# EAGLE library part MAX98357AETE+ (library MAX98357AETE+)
MAXIM INTEGRATED PRODUCTS - MAX98357AETE+ - AMPLIFIER, CLASS-D, 1-CH, 3.2W, TQFN-16 Source: Datasheet
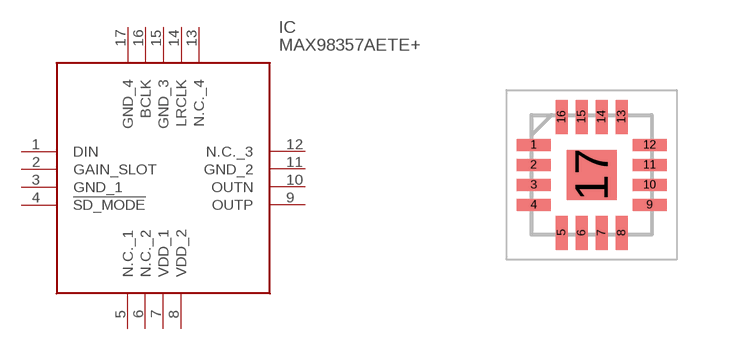
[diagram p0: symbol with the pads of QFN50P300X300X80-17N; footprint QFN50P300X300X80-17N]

Designator prefix IC

## MAX98357AETE+ (Description: MAXIM INTEGRATED PRODUCTS - MAX98357AETE+ - AMPLIFIER, CLASS-D, 1-CH, 3.2W, TQFN-16; Height: 0.8mm; Manufacturer_Name: Analog Devices; Manufacturer_Part_Number: MAX98357AETE+; Mouser_Part_Number: 700-MAX98357AETE+; Mouser_Price-Stock: https://www.mouser.co.uk/ProductDetail/Analog-Devices-Maxim-Integrated/MAX98357AETE%2b?qs=AAveGqk956EyS6m3AmZeuw%3D%3D)  [QFN50P300X300X80-17N]
1  DIN
2  GAIN_SLOT
3  GND_1
4  !SD_MODE
5  N.C._1
6  N.C._2
7  VDD_1
8  VDD_2
9  OUTP
10  OUTN
11  GND_2
12  N.C._3
13  N.C._4
14  LRCLK
15  GND_3
16  BCLK
17  GND_4

## Footprint QFN50P300X300X80-17N (pad centres in mm)
MAX98357AETE+
smd 0.85 x 0.3: 1 -1.45,0.75; 2 -1.45,0.25; 3 -1.45,-0.25; 4 -1.45,-0.75; 9 1.45,-0.75; 10 1.45,-0.25; 11 1.45,0.25; 12 1.45,0.75
smd 0.3 x 0.85: 5 -0.75,-1.45; 6 -0.25,-1.45; 7 0.25,-1.45; 8 0.75,-1.45; 13 0.75,1.45; 14 0.25,1.45; 15 -0.25,1.45; 16 -0.75,1.45
smd 1.25 x 1.25: 17 0,0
